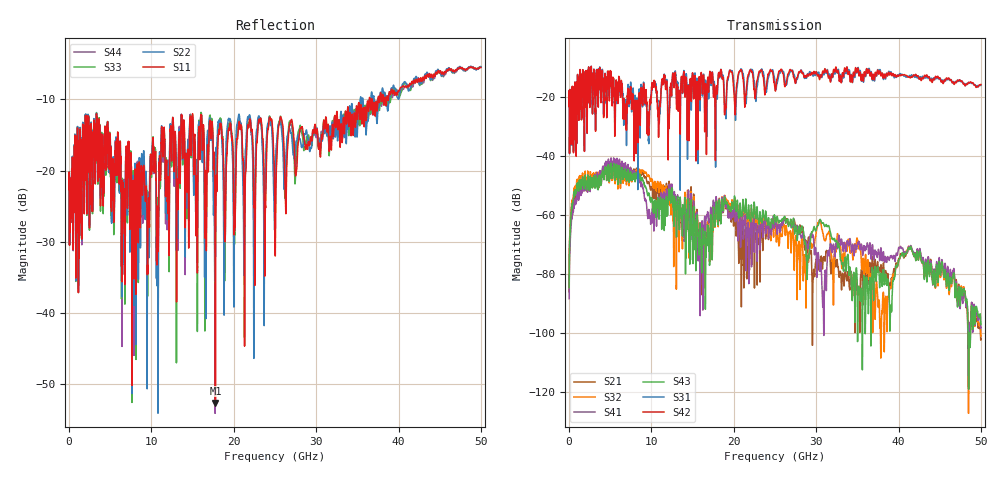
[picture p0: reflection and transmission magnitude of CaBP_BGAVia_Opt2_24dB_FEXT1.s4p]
!* Samtec Inc. NovaRay Examax Flyover System  *
!*  REV DATE  = 08/08/18  *
!*  TYPE  = TOUCHSTONE  *
!*  PORTS  = 4 port  *
!*  UNITS  = GHz  *
!*  DATA RANGE = DC  to 50 GHz; 10 MHz Step  *
!*  PARAMETER  = S  *
!*  FORMAT  = Real-Imaginary  *
!*  REFERENCE  = 50 ohms  *
!*  SOURCE  = HFSS  *
!*  VALIDATED  = No  *
!*  MANUFACTURER = SAMTEC  *
!*  INTERCONNECT = NVAx to EBCx to EBCx to NVAx  *
!*  [Full Channel NVAx to EBCx to EBCx to NVAx  with PCB Trace and BGA Via]  *
!*  BOUNDARY A  = Silicon BGA Ball Pad  *
!*  BOUNDARY B  = Silicon BGA Ball Pad  *
!*  NVAx (end a) ->>- (end b) NVAx  *
!*  Port 01 ->>- Port 02  *
!*  Port 03 ->>- Port 04  *
!***************************** CHANNEL MODEL ******************************************
# GHz S RI R 50
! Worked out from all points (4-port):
!   5000 points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, 10 MHz to 50 GHz, reference 50 ohm
!   strongest paths, dB at 10 MHz, 12.51 GHz, 25.01 GHz, 37.51 GHz, 50 GHz:
!     S42: -23.1, -14.3, -17.6, -11.1, -15.7
!     S31: -23.2, -14.5, -15.2, -10.7, -16.0
!     S43: -84.5, -53.7, -60.8, -78.5, -97.0
!     S41: -88.3, -51.6, -62.4, -72.7, -98.1
!     S32: -83.2, -56.3, -62.8, -90.1, -100.9
!     S21: -85.9, -53.8, -60.9, -76.9, -101.8
!   lowest |S11| = -52.7 dB at 17.77 GHz (marker M1), VSWR 1.00, Z = 49.8 - j0.145 ohm
!   |S11| at or under -10 dB: start of sweep to 36.46 GHz; 36.55 GHz to 36.75 GHz (204 MHz wide, 0.557 % of centre); 36.79 GHz to 37.51 GHz (722.9 MHz wide, 1.95 % of centre)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
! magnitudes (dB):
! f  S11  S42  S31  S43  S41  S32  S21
! 10 MHz  -22.7  -23.1  -23.2  -84.5  -88.3  -83.2  -85.9
! 790 MHz  -17.2  -17.6  -17.7  -52.6  -55.8  -51.4  -53.9
! 5.26 GHz  -18.9  -16.8  -16.1  -46.8  -43.9  -47.8  -45.3
! 14.64 GHz  -14.5  -17.5  -20.5  -67.6  -61.6  -66.1  -59.2
! 16.21 GHz  -16.4  -18.6  -19.4  -64.3  -69.2  -65.4  -67.1
! 17.77 GHz  -52.7  -41.5  -28.1  -61.1  -56.0  -61.7  -58.9
! 50 GHz  -5.5  -15.7  -16.0  -97.0  -98.1  -100.9  -101.8
